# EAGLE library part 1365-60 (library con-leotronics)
DUAL ROW STRAIGHT HEADER 1364 SERIES. 1.27mm x 1.27mm. Without Fixing Post. SMT Source: http://www.leotronics.co.uk/Conexcon/Data%20Sheets/sec.%20A/1364ing.pdf
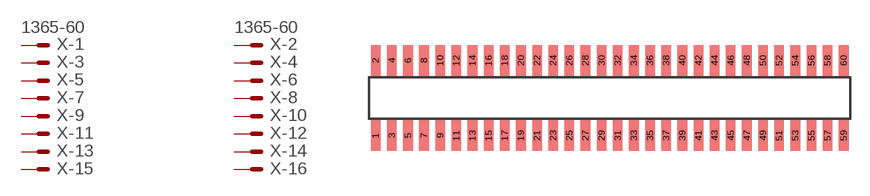
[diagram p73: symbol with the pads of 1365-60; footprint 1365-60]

Designator prefix X; gates -1=MVAL -2=MVAL -3=M -4=M -5=M -6=M -7=M -8=M -9=M -10=M -11=M -12=M -13=M -14=M -15=M -16=M -17=M -18=M -19=M -20=M -21=M -22=M -23=M -24=M -25=M -26=M -27=M -28=M -29=M -30=M -31=M -32=M -33=M -34=M -35=M -36=M -37=M -38=M -39=M -40=M -41=M -42=M -43=M -44=M -45=M -46=M -47=M -48=M -49=M -50=M -51=M -52=M -53=M -54=M -55=M -56=M -57=M -58=M -59=M -60=M

## 1365-60 (OC_FARNELL: unknown; OC_NEWARK: unknown)  [1365-60]
1  -1:S  pas
2  -2:S  pas
3  -3:S  pas
4  -4:S  pas
5  -5:S  pas
6  -6:S  pas
7  -7:S  pas
8  -8:S  pas
9  -9:S  pas
10  -10:S  pas
11  -11:S  pas
12  -12:S  pas
13  -13:S  pas
14  -14:S  pas
15  -15:S  pas
16  -16:S  pas
17  -17:S  pas
18  -18:S  pas
19  -19:S  pas
20  -20:S  pas
21  -21:S  pas
22  -22:S  pas
23  -23:S  pas
24  -24:S  pas
25  -25:S  pas
26  -26:S  pas
27  -27:S  pas
28  -28:S  pas
29  -29:S  pas
30  -30:S  pas
31  -31:S  pas
32  -32:S  pas
33  -33:S  pas
34  -34:S  pas
35  -35:S  pas
36  -36:S  pas
37  -37:S  pas
38  -38:S  pas
39  -39:S  pas
40  -40:S  pas
41  -41:S  pas
42  -42:S  pas
43  -43:S  pas
44  -44:S  pas
45  -45:S  pas
46  -46:S  pas
47  -47:S  pas
48  -48:S  pas
49  -49:S  pas
50  -50:S  pas
51  -51:S  pas
52  -52:S  pas
53  -53:S  pas
54  -54:S  pas
55  -55:S  pas
56  -56:S  pas
57  -57:S  pas
58  -58:S  pas
59  -59:S  pas
60  -60:S  pas

## Footprint 1365-60 (pad centres in mm)
DUAL ROW STRAIGHT HEADER 1364 SERIES. 1.27mm x 1.27mm. Without Fixing Post. SMT Source: http://www.leotronics.co.uk/Conexcon/Data%20Sheets/sec.%20A/1364ing.pdf
smd 0.76 x 2.4: 1 -18.415,-2.95; 2 -18.415,2.95; 3 -17.145,-2.95; 4 -17.145,2.95; 5 -15.875,-2.95; 6 -15.875,2.95; 7 -14.605,-2.95; 8 -14.605,2.95; 9 -13.335,-2.95; 10 -13.335,2.95; 11 -12.065,-2.95; 12 -12.065,2.95; 13 -10.795,-2.95; 14 -10.795,2.95; 15 -9.525,-2.95; 16 -9.525,2.95; 17 -8.255,-2.95; 18 -8.255,2.95; 19 -6.985,-2.95; 20 -6.985,2.95; 21 -5.715,-2.95; 22 -5.715,2.95; 23 -4.445,-2.95; 24 -4.445,2.95; 25 -3.175,-2.95; 26 -3.175,2.95; 27 -1.905,-2.95; 28 -1.905,2.95; 29 -0.635,-2.95; 30 -0.635,2.95; 31 0.635,-2.95; 32 0.635,2.95; 33 1.905,-2.95; 34 1.905,2.95; 35 3.175,-2.95; 36 3.175,2.95; 37 4.445,-2.95; 38 4.445,2.95; 39 5.715,-2.95; 40 5.715,2.95; 41 6.985,-2.95; 42 6.985,2.95; 43 8.255,-2.95; 44 8.255,2.95; 45 9.525,-2.95; 46 9.525,2.95; 47 10.795,-2.95; 48 10.795,2.95; 49 12.065,-2.95; 50 12.065,2.95; 51 13.335,-2.95; 52 13.335,2.95; 53 14.605,-2.95; 54 14.605,2.95; 55 15.875,-2.95; 56 15.875,2.95; 57 17.145,-2.95; 58 17.145,2.95; 59 18.415,-2.95; 60 18.415,2.95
